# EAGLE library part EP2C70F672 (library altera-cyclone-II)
EP2C70F672 Auto generated by make-symbol-device-package-bsdl.ulp Rev. 19 Tip: Use split-device-symbol.ulp to generate a Device with multiple small symbols! Read HELP. Source: EP2C70F672.BSD
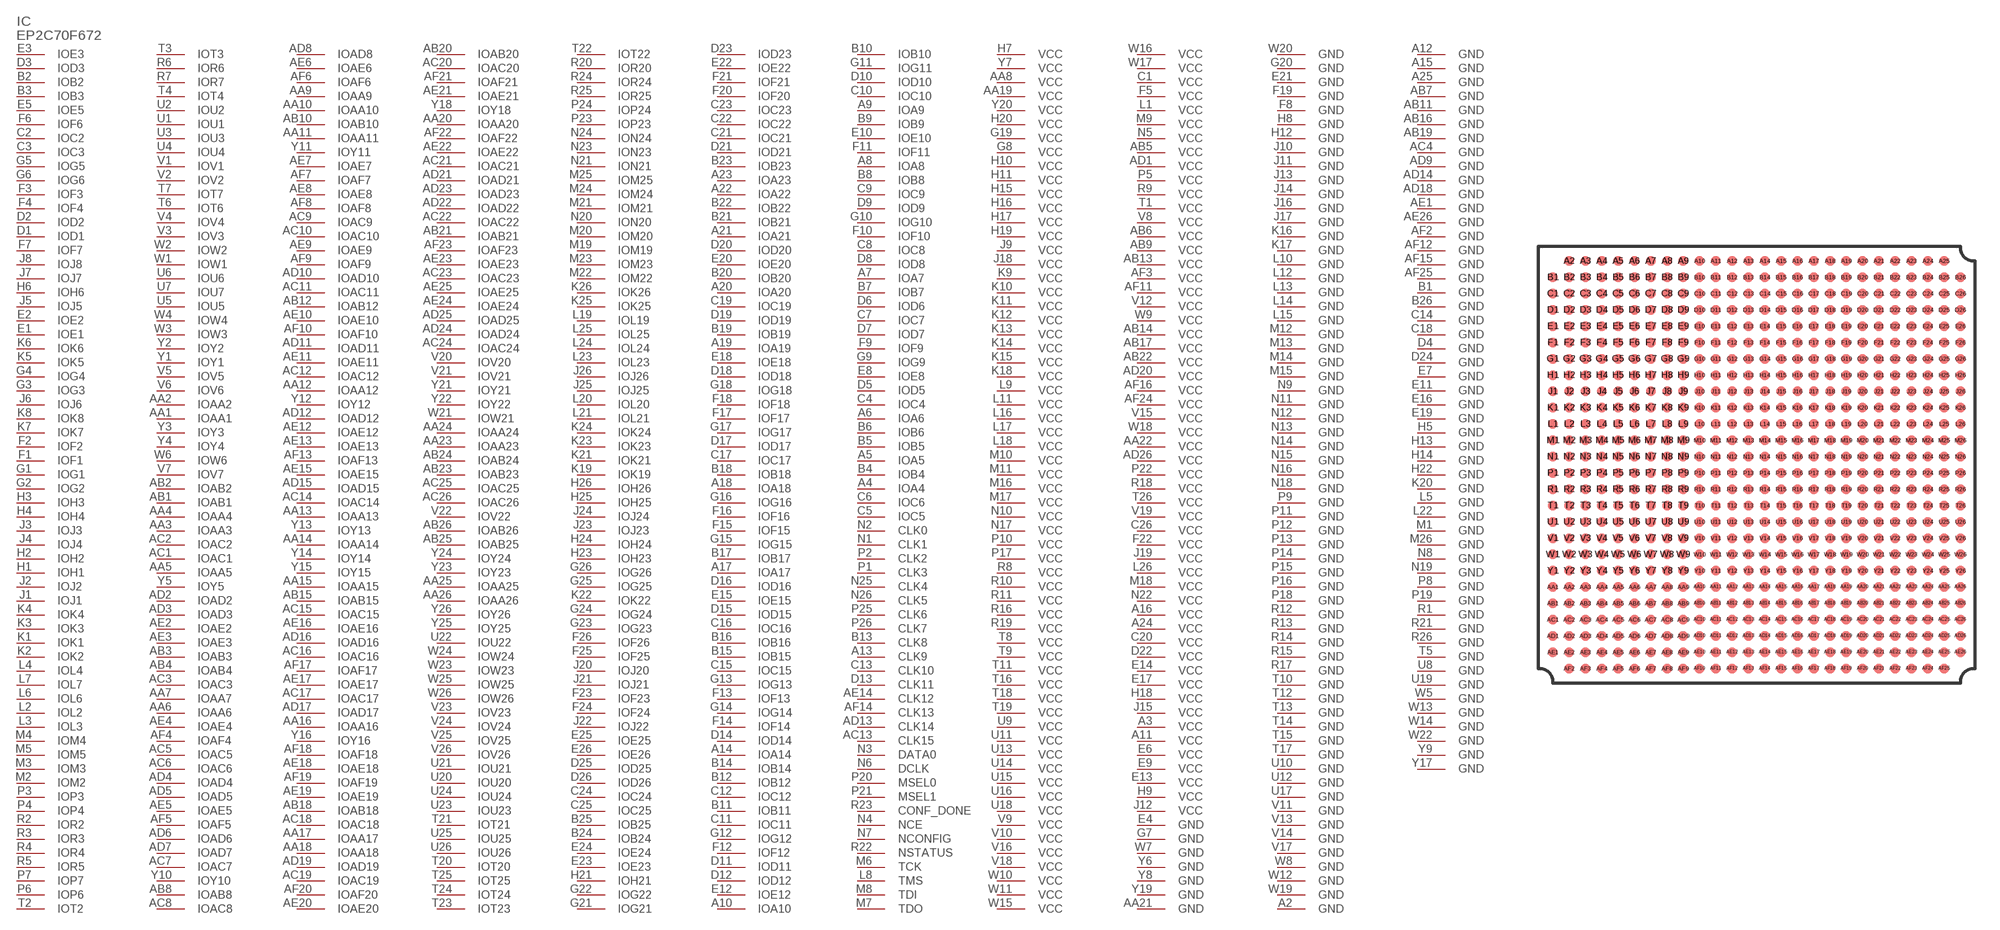
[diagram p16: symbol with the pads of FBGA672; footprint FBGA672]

Designator prefix IC

## EP2C70F672 (MPN: EP2C70F672C8N; OC_FARNELL: 1635091; OC_NEWARK: 51R0572)  [FBGA672]
A2  GND  pwr
A3  VCC  pwr
A4  IOA4
A5  IOA5
A6  IOA6
A7  IOA7
A8  IOA8
A9  IOA9
A10  IOA10
A11  VCC  pwr
A12  GND  pwr
A13  CLK9
A14  IOA14
A15  GND  pwr
A16  VCC  pwr
A17  IOA17
A18  IOA18
A19  IOA19
A20  IOA20
A21  IOA21
A22  IOA22
A23  IOA23
A24  VCC  pwr
A25  GND  pwr
AA1  IOAA1
AA2  IOAA2
AA3  IOAA3
AA4  IOAA4
AA5  IOAA5
AA6  IOAA6
AA7  IOAA7
AA8  VCC  pwr
AA9  IOAA9
AA10  IOAA10
AA11  IOAA11
AA12  IOAA12
AA13  IOAA13
AA14  IOAA14
AA15  IOAA15
AA16  IOAA16
AA17  IOAA17
AA18  IOAA18
AA19  VCC  pwr
AA20  IOAA20
AA21  GND  pwr
AA22  VCC  pwr
AA23  IOAA23
AA24  IOAA24
AA25  IOAA25
AA26  IOAA26
AB1  IOAB1
AB2  IOAB2
AB3  IOAB3
AB4  IOAB4
AB5  VCC  pwr
AB6  VCC  pwr
AB7  GND  pwr
AB8  IOAB8
AB9  VCC  pwr
AB10  IOAB10
AB11  GND  pwr
AB12  IOAB12
AB13  VCC  pwr
AB14  VCC  pwr
AB15  IOAB15
AB16  GND  pwr
AB17  VCC  pwr
AB18  IOAB18
AB19  GND  pwr
AB20  IOAB20
AB21  IOAB21
AB22  VCC  pwr
AB23  IOAB23
AB24  IOAB24
AB25  IOAB25
AB26  IOAB26
AC1  IOAC1
AC2  IOAC2
AC3  IOAC3
AC4  GND  pwr
AC5  IOAC5
AC6  IOAC6
AC7  IOAC7
AC8  IOAC8
AC9  IOAC9
AC10  IOAC10
AC11  IOAC11
AC12  IOAC12
AC13  CLK15
AC14  IOAC14
AC15  IOAC15
AC16  IOAC16
AC17  IOAC17
AC18  IOAC18
AC19  IOAC19
AC20  IOAC20
AC21  IOAC21
AC22  IOAC22
AC23  IOAC23
AC24  IOAC24
AC25  IOAC25
AC26  IOAC26
AD1  VCC  pwr
AD2  IOAD2
AD3  IOAD3
AD4  IOAD4
AD5  IOAD5
AD6  IOAD6
AD7  IOAD7
AD8  IOAD8
AD9  GND  pwr
AD10  IOAD10
AD11  IOAD11
AD12  IOAD12
AD13  CLK14
AD14  GND  pwr
AD15  IOAD15
AD16  IOAD16
AD17  IOAD17
AD18  GND  pwr
AD19  IOAD19
AD20  VCC  pwr
AD21  IOAD21
AD22  IOAD22
AD23  IOAD23
AD24  IOAD24
AD25  IOAD25
AD26  VCC  pwr
AE1  GND  pwr
AE2  IOAE2
AE3  IOAE3
AE4  IOAE4
AE5  IOAE5
AE6  IOAE6
AE7  IOAE7
AE8  IOAE8
AE9  IOAE9
AE10  IOAE10
AE11  IOAE11
AE12  IOAE12
AE13  IOAE13
AE14  CLK12
AE15  IOAE15
AE16  IOAE16
AE17  IOAE17
AE18  IOAE18
AE19  IOAE19
AE20  IOAE20
AE21  IOAE21
AE22  IOAE22
AE23  IOAE23
AE24  IOAE24
AE25  IOAE25
AE26  GND  pwr
AF2  GND  pwr
AF3  VCC  pwr
AF4  IOAF4
AF5  IOAF5
AF6  IOAF6
AF7  IOAF7
AF8  IOAF8
AF9  IOAF9
AF10  IOAF10
AF11  VCC  pwr
AF12  GND  pwr
AF13  IOAF13
AF14  CLK13
AF15  GND  pwr
AF16  VCC  pwr
AF17  IOAF17
AF18  IOAF18
AF19  IOAF19
AF20  IOAF20
AF21  IOAF21
AF22  IOAF22
AF23  IOAF23
AF24  VCC  pwr
AF25  GND  pwr
B1  GND  pwr
B2  IOB2
B3  IOB3
B4  IOB4
B5  IOB5
B6  IOB6
B7  IOB7
B8  IOB8
B9  IOB9
B10  IOB10
B11  IOB11
B12  IOB12
B13  CLK8
B14  IOB14
B15  IOB15
B16  IOB16
B17  IOB17
B18  IOB18
B19  IOB19
B20  IOB20
B21  IOB21
B22  IOB22
B23  IOB23
B24  IOB24
B25  IOB25
B26  GND  pwr
C1  VCC  pwr
C2  IOC2
C3  IOC3
C4  IOC4
C5  IOC5
C6  IOC6
C7  IOC7
C8  IOC8
C9  IOC9
C10  IOC10
C11  IOC11
C12  IOC12
C13  CLK10
C14  GND  pwr
C15  IOC15
C16  IOC16
C17  IOC17
C18  GND  pwr
C19  IOC19
C20  VCC  pwr
C21  IOC21
C22  IOC22
C23  IOC23
C24  IOC24
C25  IOC25
C26  VCC  pwr
D1  IOD1
D2  IOD2
D3  IOD3  out
D4  GND  pwr
D5  IOD5
D6  IOD6
D7  IOD7
D8  IOD8
D9  IOD9
D10  IOD10
D11  IOD11
D12  IOD12
D13  CLK11
D14  IOD14
D15  IOD15
D16  IOD16
D17  IOD17
D18  IOD18
D19  IOD19
D20  IOD20
D21  IOD21
D22  VCC  pwr
D23  IOD23
D24  GND  pwr
D25  IOD25
D26  IOD26
E1  IOE1
E2  IOE2
E3  IOE3  out
E4  GND  pwr
E5  IOE5
E6  VCC  pwr
E7  GND  pwr
E8  IOE8
E9  VCC  pwr
E10  IOE10
E11  GND  pwr
E12  IOE12
E13  VCC  pwr
E14  VCC  pwr
E15  IOE15
E16  GND  pwr
E17  VCC  pwr
E18  IOE18
E19  GND  pwr
E20  IOE20
E21  GND  pwr
E22  IOE22
E23  IOE23
E24  IOE24
E25  IOE25
E26  IOE26
F1  IOF1
F2  IOF2
F3  IOF3
F4  IOF4
F5  VCC  pwr
F6  IOF6
F7  IOF7
F8  GND  pwr
F9  IOF9
F10  IOF10
F11  IOF11
F12  IOF12
F13  IOF13
F14  IOF14
F15  IOF15
F16  IOF16
F17  IOF17
F18  IOF18
F19  GND  pwr
F20  IOF20
F21  IOF21
F22  VCC  pwr
F23  IOF23
F24  IOF24
F25  IOF25
F26  IOF26
G1  IOG1
G2  IOG2
G3  IOG3
G4  IOG4
G5  IOG5
G6  IOG6
G7  GND  pwr
G8  VCC  pwr
G9  IOG9
G10  IOG10
G11  IOG11
G12  IOG12
G13  IOG13
G14  IOG14
G15  IOG15
G16  IOG16
G17  IOG17
G18  IOG18
G19  VCC  pwr
G20  GND  pwr
G21  IOG21
G22  IOG22
G23  IOG23
G24  IOG24
G25  IOG25
G26  IOG26
H1  IOH1
H2  IOH2
H3  IOH3
H4  IOH4
H5  GND  pwr
H6  IOH6
H7  VCC  pwr
H8  GND  pwr
H9  VCC  pwr
H10  VCC  pwr
H11  VCC  pwr
H12  GND  pwr
H13  GND  pwr
H14  GND  pwr
H15  VCC  pwr
H16  VCC  pwr
H17  VCC  pwr
H18  VCC  pwr
H19  VCC  pwr
H20  VCC  pwr
H21  IOH21
H22  GND  pwr
H23  IOH23
H24  IOH24
H25  IOH25
H26  IOH26
J1  IOJ1
J2  IOJ2
J3  IOJ3
J4  IOJ4
J5  IOJ5
J6  IOJ6
J7  IOJ7
J8  IOJ8
J9  VCC  pwr
J10  GND  pwr
J11  GND  pwr
J12  VCC  pwr
J13  GND  pwr
J14  GND  pwr
J15  VCC  pwr
J16  GND  pwr
J17  GND  pwr
J18  VCC  pwr
J19  VCC  pwr
J20  IOJ20
J21  IOJ21
J22  IOJ22
J23  IOJ23
J24  IOJ24
J25  IOJ25
J26  IOJ26
K1  IOK1
K2  IOK2
K3  IOK3
K4  IOK4
K5  IOK5
K6  IOK6
K7  IOK7
K8  IOK8
K9  VCC  pwr
K10  VCC  pwr
K11  VCC  pwr
K12  VCC  pwr
K13  VCC  pwr
K14  VCC  pwr
K15  VCC  pwr
K16  GND  pwr
K17  GND  pwr
K18  VCC  pwr
K19  IOK19
K20  GND  pwr
K21  IOK21
K22  IOK22
K23  IOK23
K24  IOK24
K25  IOK25
K26  IOK26
L1  VCC  pwr
L2  IOL2
L3  IOL3
L4  IOL4
L5  GND  pwr
L6  IOL6
L7  IOL7
L8  TMS  in
L9  VCC  pwr
L10  GND  pwr
L11  VCC  pwr
L12  GND  pwr
L13  GND  pwr
L14  GND  pwr
L15  GND  pwr
L16  VCC  pwr
L17  VCC  pwr
L18  VCC  pwr
L19  IOL19
L20  IOL20
L21  IOL21
L22  GND  pwr
L23  IOL23
L24  IOL24
L25  IOL25
L26  VCC  pwr
M1  GND  pwr
M2  IOM2
M3  IOM3
M4  IOM4
M5  IOM5
M6  TCK  in
M7  TDO  out
M8  TDI  in
M9  VCC  pwr
M10  VCC  pwr
M11  VCC  pwr
M12  GND  pwr
M13  GND  pwr
M14  GND  pwr
M15  GND  pwr
M16  VCC  pwr
M17  VCC  pwr
M18  VCC  pwr
M19  IOM19
M20  IOM20
M21  IOM21
M22  IOM22
M23  IOM23
M24  IOM24
M25  IOM25
M26  GND  pwr
N1  CLK1
N2  CLK0
N3  DATA0
N4  NCE  in
N5  VCC  pwr
N6  DCLK
N7  NCONFIG  in
N8  GND  pwr
N9  GND  pwr
N10  VCC  pwr
N11  GND  pwr
N12  GND  pwr
N13  GND  pwr
N14  GND  pwr
N15  GND  pwr
N16  GND  pwr
N17  VCC  pwr
N18  GND  pwr
N19  GND  pwr
N20  ION20
N21  ION21
N22  VCC  pwr
N23  ION23
N24  ION24
N25  CLK4
N26  CLK5
P1  CLK3
P2  CLK2
P3  IOP3
P4  IOP4
P5  VCC  pwr
P6  IOP6
P7  IOP7
P8  GND  pwr
P9  GND  pwr
P10  VCC  pwr
P11  GND  pwr
P12  GND  pwr
P13  GND  pwr
P14  GND  pwr
P15  GND  pwr
P16  GND  pwr
P17  VCC  pwr
P18  GND  pwr
P19  GND  pwr
P20  MSEL0  in
P21  MSEL1  in
P22  VCC  pwr
P23  IOP23
P24  IOP24
P25  CLK6
P26  CLK7
R1  GND  pwr
R2  IOR2
R3  IOR3
R4  IOR4
R5  IOR5
R6  IOR6
R7  IOR7
R8  VCC  pwr
R9  VCC  pwr
R10  VCC  pwr
R11  VCC  pwr
R12  GND  pwr
R13  GND  pwr
R14  GND  pwr
R15  GND  pwr
R16  VCC  pwr
R17  GND  pwr
R18  VCC  pwr
R19  VCC  pwr
R20  IOR20
R21  GND  pwr
R22  NSTATUS  in
R23  CONF_DONE  in
R24  IOR24
R25  IOR25
R26  GND  pwr
T1  VCC  pwr
T2  IOT2
T3  IOT3
T4  IOT4
T5  GND  pwr
T6  IOT6
T7  IOT7
T8  VCC  pwr
T9  VCC  pwr
T10  GND  pwr
T11  VCC  pwr
T12  GND  pwr
T13  GND  pwr
T14  GND  pwr
T15  GND  pwr
T16  VCC  pwr
T17  GND  pwr
T18  VCC  pwr
T19  VCC  pwr
T20  IOT20
T21  IOT21
T22  IOT22
T23  IOT23
T24  IOT24
T25  IOT25
T26  VCC  pwr
U1  IOU1
U2  IOU2
U3  IOU3
U4  IOU4
U5  IOU5
U6  IOU6
U7  IOU7
U8  GND  pwr
U9  VCC  pwr
U10  GND  pwr
U11  VCC  pwr
U12  GND  pwr
U13  VCC  pwr
U14  VCC  pwr
U15  VCC  pwr
U16  VCC  pwr
U17  GND  pwr
U18  VCC  pwr
U19  GND  pwr
U20  IOU20
U21  IOU21
U22  IOU22
U23  IOU23
U24  IOU24
U25  IOU25
U26  IOU26
V1  IOV1
V2  IOV2
V3  IOV3
V4  IOV4
V5  IOV5
V6  IOV6
V7  IOV7
V8  VCC  pwr
V9  VCC  pwr
V10  VCC  pwr
V11  GND  pwr
V12  VCC  pwr
V13  GND  pwr
V14  GND  pwr
V15  VCC  pwr
V16  VCC  pwr
V17  GND  pwr
V18  VCC  pwr
V19  VCC  pwr
V20  IOV20
V21  IOV21
V22  IOV22
V23  IOV23
V24  IOV24
V25  IOV25
V26  IOV26
W1  IOW1
W2  IOW2
W3  IOW3
W4  IOW4
W5  GND  pwr
W6  IOW6
W7  GND  pwr
W8  GND  pwr
W9  VCC  pwr
W10  VCC  pwr
W11  VCC  pwr
W12  GND  pwr
W13  GND  pwr
W14  GND  pwr
W15  VCC  pwr
W16  VCC  pwr
W17  VCC  pwr
W18  VCC  pwr
W19  GND  pwr
W20  GND  pwr
W21  IOW21
W22  GND  pwr
W23  IOW23
W24  IOW24
W25  IOW25
W26  IOW26
Y1  IOY1
Y2  IOY2
Y3  IOY3
Y4  IOY4
Y5  IOY5
Y6  GND  pwr
Y7  VCC  pwr
Y8  GND  pwr
Y9  GND  pwr
Y10  IOY10
Y11  IOY11
Y12  IOY12
Y13  IOY13
Y14  IOY14
Y15  IOY15
Y16  IOY16
Y17  GND  pwr
Y18  IOY18
Y19  GND  pwr
Y20  VCC  pwr
Y21  IOY21
Y22  IOY22
Y23  IOY23
Y24  IOY24
Y25  IOY25
Y26  IOY26

## Footprint FBGA672 (pad centres in mm)
EP2C35F672 Auto generated by make-symbol-device-package-bsdl.ulp Rev. 19 Source: EP2C35F672.BSD www.altera.com .. cyc2_cii51015.pdf
smd 0.6 x 0.6: A2 -11.5,12.5; A3 -10.5,12.5; A4 -9.5,12.5; A5 -8.5,12.5; A6 -7.5,12.5; A7 -6.5,12.5; A8 -5.5,12.5; A9 -4.5,12.5; A10 -3.5,12.5; A11 -2.5,12.5; A12 -1.5,12.5; A13 -0.5,12.5; A14 0.5,12.5; A15 1.5,12.5; A16 2.5,12.5; A17 3.5,12.5; A18 4.5,12.5; A19 5.5,12.5; A20 6.5,12.5; A21 7.5,12.5; A22 8.5,12.5; A23 9.5,12.5; A24 10.5,12.5; A25 11.5,12.5; AA1 -12.5,-7.5; AA2 -11.5,-7.5; AA3 -10.5,-7.5; AA4 -9.5,-7.5; AA5 -8.5,-7.5; AA6 -7.5,-7.5; AA7 -6.5,-7.5; AA8 -5.5,-7.5; AA9 -4.5,-7.5; AA10 -3.5,-7.5; AA11 -2.5,-7.5; AA12 -1.5,-7.5; AA13 -0.5,-7.5; AA14 0.5,-7.5; AA15 1.5,-7.5; AA16 2.5,-7.5; AA17 3.5,-7.5; AA18 4.5,-7.5; AA19 5.5,-7.5; AA20 6.5,-7.5; AA21 7.5,-7.5; AA22 8.5,-7.5; AA23 9.5,-7.5; AA24 10.5,-7.5; AA25 11.5,-7.5; AA26 12.5,-7.5; AB1 -12.5,-8.5; AB2 -11.5,-8.5; AB3 -10.5,-8.5; AB4 -9.5,-8.5; AB5 -8.5,-8.5; AB6 -7.5,-8.5; AB7 -6.5,-8.5; AB8 -5.5,-8.5; AB9 -4.5,-8.5; AB10 -3.5,-8.5; AB11 -2.5,-8.5; AB12 -1.5,-8.5; AB13 -0.5,-8.5; AB14 0.5,-8.5; AB15 1.5,-8.5; AB16 2.5,-8.5; AB17 3.5,-8.5; AB18 4.5,-8.5; AB19 5.5,-8.5; AB20 6.5,-8.5; AB21 7.5,-8.5; AB22 8.5,-8.5; AB23 9.5,-8.5; AB24 10.5,-8.5; AB25 11.5,-8.5; AB26 12.5,-8.5; AC1 -12.5,-9.5; AC2 -11.5,-9.5; AC3 -10.5,-9.5; AC4 -9.5,-9.5; AC5 -8.5,-9.5; AC6 -7.5,-9.5; AC7 -6.5,-9.5; AC8 -5.5,-9.5; AC9 -4.5,-9.5; AC10 -3.5,-9.5; AC11 -2.5,-9.5; AC12 -1.5,-9.5; AC13 -0.5,-9.5; AC14 0.5,-9.5; AC15 1.5,-9.5; AC16 2.5,-9.5; AC17 3.5,-9.5; AC18 4.5,-9.5; AC19 5.5,-9.5; AC20 6.5,-9.5; AC21 7.5,-9.5; AC22 8.5,-9.5; AC23 9.5,-9.5; AC24 10.5,-9.5; AC25 11.5,-9.5; AC26 12.5,-9.5; AD1 -12.5,-10.5; AD2 -11.5,-10.5; AD3 -10.5,-10.5; AD4 -9.5,-10.5; AD5 -8.5,-10.5; AD6 -7.5,-10.5; AD7 -6.5,-10.5; AD8 -5.5,-10.5; AD9 -4.5,-10.5; AD10 -3.5,-10.5; AD11 -2.5,-10.5; AD12 -1.5,-10.5; AD13 -0.5,-10.5; AD14 0.5,-10.5; AD15 1.5,-10.5; AD16 2.5,-10.5; AD17 3.5,-10.5; AD18 4.5,-10.5; AD19 5.5,-10.5; AD20 6.5,-10.5; AD21 7.5,-10.5; AD22 8.5,-10.5; AD23 9.5,-10.5; AD24 10.5,-10.5; AD25 11.5,-10.5; AD26 12.5,-10.5; AE1 -12.5,-11.5; AE2 -11.5,-11.5; AE3 -10.5,-11.5; AE4 -9.5,-11.5; AE5 -8.5,-11.5; AE6 -7.5,-11.5; AE7 -6.5,-11.5; AE8 -5.5,-11.5; AE9 -4.5,-11.5; AE10 -3.5,-11.5; AE11 -2.5,-11.5; AE12 -1.5,-11.5; AE13 -0.5,-11.5; AE14 0.5,-11.5; AE15 1.5,-11.5; AE16 2.5,-11.5; AE17 3.5,-11.5; AE18 4.5,-11.5; AE19 5.5,-11.5; AE20 6.5,-11.5; AE21 7.5,-11.5; AE22 8.5,-11.5; AE23 9.5,-11.5; AE24 10.5,-11.5; AE25 11.5,-11.5; AE26 12.5,-11.5; AF2 -11.5,-12.5; AF3 -10.5,-12.5; AF4 -9.5,-12.5; AF5 -8.5,-12.5; AF6 -7.5,-12.5; AF7 -6.5,-12.5; AF8 -5.5,-12.5; AF9 -4.5,-12.5; AF10 -3.5,-12.5; AF11 -2.5,-12.5; AF12 -1.5,-12.5; AF13 -0.5,-12.5; AF14 0.5,-12.5; AF15 1.5,-12.5; AF16 2.5,-12.5; AF17 3.5,-12.5; AF18 4.5,-12.5; AF19 5.5,-12.5; AF20 6.5,-12.5; AF21 7.5,-12.5; AF22 8.5,-12.5; AF23 9.5,-12.5; AF24 10.5,-12.5; AF25 11.5,-12.5; B1 -12.5,11.5; B2 -11.5,11.5; B3 -10.5,11.5; B4 -9.5,11.5; B5 -8.5,11.5; B6 -7.5,11.5; B7 -6.5,11.5; B8 -5.5,11.5; B9 -4.5,11.5; B10 -3.5,11.5; B11 -2.5,11.5; B12 -1.5,11.5; B13 -0.5,11.5; B14 0.5,11.5; B15 1.5,11.5; B16 2.5,11.5; B17 3.5,11.5; B18 4.5,11.5; B19 5.5,11.5; B20 6.5,11.5; B21 7.5,11.5; B22 8.5,11.5; B23 9.5,11.5; B24 10.5,11.5; B25 11.5,11.5; B26 12.5,11.5; C1 -12.5,10.5; C2 -11.5,10.5; C3 -10.5,10.5; C4 -9.5,10.5; C5 -8.5,10.5; C6 -7.5,10.5; C7 -6.5,10.5; C8 -5.5,10.5; C9 -4.5,10.5; C10 -3.5,10.5; C11 -2.5,10.5; C12 -1.5,10.5; C13 -0.5,10.5; C14 0.5,10.5; C15 1.5,10.5; C16 2.5,10.5; C17 3.5,10.5; C18 4.5,10.5; C19 5.5,10.5; C20 6.5,10.5; C21 7.5,10.5; C22 8.5,10.5; C23 9.5,10.5; C24 10.5,10.5; C25 11.5,10.5; C26 12.5,10.5; D1 -12.5,9.5; D2 -11.5,9.5; D3 -10.5,9.5; D4 -9.5,9.5; D5 -8.5,9.5; D6 -7.5,9.5; D7 -6.5,9.5; D8 -5.5,9.5; D9 -4.5,9.5; D10 -3.5,9.5; D11 -2.5,9.5; D12 -1.5,9.5; D13 -0.5,9.5; D14 0.5,9.5; D15 1.5,9.5; D16 2.5,9.5; D17 3.5,9.5; D18 4.5,9.5; D19 5.5,9.5; D20 6.5,9.5; D21 7.5,9.5; D22 8.5,9.5; D23 9.5,9.5; D24 10.5,9.5; D25 11.5,9.5; D26 12.5,9.5; E1 -12.5,8.5; E2 -11.5,8.5; E3 -10.5,8.5; E4 -9.5,8.5; E5 -8.5,8.5; E6 -7.5,8.5; E7 -6.5,8.5; E8 -5.5,8.5; E9 -4.5,8.5; E10 -3.5,8.5; E11 -2.5,8.5; E12 -1.5,8.5; E13 -0.5,8.5; E14 0.5,8.5; E15 1.5,8.5; E16 2.5,8.5; E17 3.5,8.5; E18 4.5,8.5; E19 5.5,8.5; E20 6.5,8.5; E21 7.5,8.5; E22 8.5,8.5; E23 9.5,8.5; E24 10.5,8.5; E25 11.5,8.5; E26 12.5,8.5; F1 -12.5,7.5; F2 -11.5,7.5; F3 -10.5,7.5; F4 -9.5,7.5; F5 -8.5,7.5; F6 -7.5,7.5; F7 -6.5,7.5; F8 -5.5,7.5; F9 -4.5,7.5; F10 -3.5,7.5; F11 -2.5,7.5; F12 -1.5,7.5; F13 -0.5,7.5; F14 0.5,7.5; F15 1.5,7.5; F16 2.5,7.5; F17 3.5,7.5; F18 4.5,7.5; F19 5.5,7.5; F20 6.5,7.5; F21 7.5,7.5; F22 8.5,7.5; F23 9.5,7.5; F24 10.5,7.5; F25 11.5,7.5; F26 12.5,7.5; G1 -12.5,6.5; G2 -11.5,6.5; G3 -10.5,6.5; G4 -9.5,6.5; G5 -8.5,6.5; G6 -7.5,6.5; G7 -6.5,6.5; G8 -5.5,6.5; G9 -4.5,6.5; G10 -3.5,6.5; G11 -2.5,6.5; G12 -1.5,6.5; G13 -0.5,6.5; G14 0.5,6.5; G15 1.5,6.5; G16 2.5,6.5; G17 3.5,6.5; G18 4.5,6.5; G19 5.5,6.5; G20 6.5,6.5; G21 7.5,6.5; G22 8.5,6.5; G23 9.5,6.5; G24 10.5,6.5; G25 11.5,6.5; G26 12.5,6.5; H1 -12.5,5.5; H2 -11.5,5.5; H3 -10.5,5.5; H4 -9.5,5.5; H5 -8.5,5.5; H6 -7.5,5.5; H7 -6.5,5.5; H8 -5.5,5.5; H9 -4.5,5.5; H10 -3.5,5.5; H11 -2.5,5.5; H12 -1.5,5.5; H13 -0.5,5.5; H14 0.5,5.5; H15 1.5,5.5; H16 2.5,5.5; H17 3.5,5.5; H18 4.5,5.5; H19 5.5,5.5; H20 6.5,5.5; H21 7.5,5.5; H22 8.5,5.5; H23 9.5,5.5; H24 10.5,5.5; H25 11.5,5.5; H26 12.5,5.5; J1 -12.5,4.5; J2 -11.5,4.5; J3 -10.5,4.5; J4 -9.5,4.5; J5 -8.5,4.5; J6 -7.5,4.5; J7 -6.5,4.5; J8 -5.5,4.5; J9 -4.5,4.5; J10 -3.5,4.5; J11 -2.5,4.5; J12 -1.5,4.5; J13 -0.5,4.5; J14 0.5,4.5; J15 1.5,4.5; J16 2.5,4.5; J17 3.5,4.5; J18 4.5,4.5; J19 5.5,4.5; J20 6.5,4.5; J21 7.5,4.5; J22 8.5,4.5; J23 9.5,4.5; J24 10.5,4.5; J25 11.5,4.5; J26 12.5,4.5; K1 -12.5,3.5; K2 -11.5,3.5; K3 -10.5,3.5; K4 -9.5,3.5; K5 -8.5,3.5; K6 -7.5,3.5; K7 -6.5,3.5; K8 -5.5,3.5; K9 -4.5,3.5; K10 -3.5,3.5; K11 -2.5,3.5; K12 -1.5,3.5; K13 -0.5,3.5; K14 0.5,3.5; K15 1.5,3.5; K16 2.5,3.5; K17 3.5,3.5; K18 4.5,3.5; K19 5.5,3.5; K20 6.5,3.5; K21 7.5,3.5; K22 8.5,3.5; K23 9.5,3.5; K24 10.5,3.5; K25 11.5,3.5; K26 12.5,3.5; L1 -12.5,2.5; L2 -11.5,2.5; L3 -10.5,2.5; L4 -9.5,2.5; L5 -8.5,2.5; L6 -7.5,2.5; L7 -6.5,2.5; L8 -5.5,2.5; L9 -4.5,2.5; L10 -3.5,2.5; L11 -2.5,2.5; L12 -1.5,2.5; L13 -0.5,2.5; L14 0.5,2.5; L15 1.5,2.5; L16 2.5,2.5; L17 3.5,2.5; L18 4.5,2.5; L19 5.5,2.5; L20 6.5,2.5; L21 7.5,2.5; L22 8.5,2.5; L23 9.5,2.5; L24 10.5,2.5; L25 11.5,2.5; L26 12.5,2.5; M1 -12.5,1.5; M2 -11.5,1.5; M3 -10.5,1.5; M4 -9.5,1.5; M5 -8.5,1.5; M6 -7.5,1.5; M7 -6.5,1.5; M8 -5.5,1.5; M9 -4.5,1.5; M10 -3.5,1.5; M11 -2.5,1.5; M12 -1.5,1.5; M13 -0.5,1.5; M14 0.5,1.5; M15 1.5,1.5; M16 2.5,1.5; M17 3.5,1.5; M18 4.5,1.5; M19 5.5,1.5; M20 6.5,1.5; M21 7.5,1.5; M22 8.5,1.5; M23 9.5,1.5; M24 10.5,1.5; M25 11.5,1.5; M26 12.5,1.5; N1 -12.5,0.5; N2 -11.5,0.5; N3 -10.5,0.5; N4 -9.5,0.5; N5 -8.5,0.5; N6 -7.5,0.5; N7 -6.5,0.5; N8 -5.5,0.5; N9 -4.5,0.5; N10 -3.5,0.5; N11 -2.5,0.5; N12 -1.5,0.5; N13 -0.5,0.5; N14 0.5,0.5; N15 1.5,0.5; N16 2.5,0.5; N17 3.5,0.5; N18 4.5,0.5; N19 5.5,0.5; N20 6.5,0.5; N21 7.5,0.5; N22 8.5,0.5; N23 9.5,0.5; N24 10.5,0.5; N25 11.5,0.5; N26 12.5,0.5; P1 -12.5,-0.5; P2 -11.5,-0.5; P3 -10.5,-0.5; P4 -9.5,-0.5; P5 -8.5,-0.5; P6 -7.5,-0.5; P7 -6.5,-0.5; P8 -5.5,-0.5; P9 -4.5,-0.5; P10 -3.5,-0.5; P11 -2.5,-0.5; P12 -1.5,-0.5; P13 -0.5,-0.5; P14 0.5,-0.5; P15 1.5,-0.5; P16 2.5,-0.5; P17 3.5,-0.5; P18 4.5,-0.5; P19 5.5,-0.5; P20 6.5,-0.5; P21 7.5,-0.5; P22 8.5,-0.5; P23 9.5,-0.5; P24 10.5,-0.5; P25 11.5,-0.5; P26 12.5,-0.5; R1 -12.5,-1.5; R2 -11.5,-1.5; R3 -10.5,-1.5; R4 -9.5,-1.5; R5 -8.5,-1.5; R6 -7.5,-1.5; R7 -6.5,-1.5; R8 -5.5,-1.5; R9 -4.5,-1.5; R10 -3.5,-1.5; R11 -2.5,-1.5; R12 -1.5,-1.5; R13 -0.5,-1.5; R14 0.5,-1.5; R15 1.5,-1.5; R16 2.5,-1.5; R17 3.5,-1.5; R18 4.5,-1.5; R19 5.5,-1.5; R20 6.5,-1.5; R21 7.5,-1.5; R22 8.5,-1.5; R23 9.5,-1.5; R24 10.5,-1.5; R25 11.5,-1.5; R26 12.5,-1.5; T1 -12.5,-2.5; T2 -11.5,-2.5; T3 -10.5,-2.5; T4 -9.5,-2.5; T5 -8.5,-2.5; T6 -7.5,-2.5; T7 -6.5,-2.5; T8 -5.5,-2.5; T9 -4.5,-2.5; T10 -3.5,-2.5; T11 -2.5,-2.5; T12 -1.5,-2.5; T13 -0.5,-2.5; T14 0.5,-2.5; T15 1.5,-2.5; T16 2.5,-2.5; T17 3.5,-2.5; T18 4.5,-2.5; T19 5.5,-2.5; T20 6.5,-2.5; T21 7.5,-2.5; T22 8.5,-2.5; T23 9.5,-2.5; T24 10.5,-2.5; T25 11.5,-2.5; T26 12.5,-2.5; U1 -12.5,-3.5; U2 -11.5,-3.5; U3 -10.5,-3.5; U4 -9.5,-3.5; U5 -8.5,-3.5; U6 -7.5,-3.5; U7 -6.5,-3.5; U8 -5.5,-3.5; U9 -4.5,-3.5; U10 -3.5,-3.5; U11 -2.5,-3.5; U12 -1.5,-3.5; U13 -0.5,-3.5; U14 0.5,-3.5; U15 1.5,-3.5; U16 2.5,-3.5; U17 3.5,-3.5; U18 4.5,-3.5; U19 5.5,-3.5; U20 6.5,-3.5; U21 7.5,-3.5; U22 8.5,-3.5; U23 9.5,-3.5; U24 10.5,-3.5; U25 11.5,-3.5; U26 12.5,-3.5; V1 -12.5,-4.5; V2 -11.5,-4.5; V3 -10.5,-4.5; V4 -9.5,-4.5; V5 -8.5,-4.5; V6 -7.5,-4.5; V7 -6.5,-4.5; V8 -5.5,-4.5; V9 -4.5,-4.5; V10 -3.5,-4.5; V11 -2.5,-4.5; V12 -1.5,-4.5; V13 -0.5,-4.5; V14 0.5,-4.5; V15 1.5,-4.5; V16 2.5,-4.5; V17 3.5,-4.5; V18 4.5,-4.5; V19 5.5,-4.5; V20 6.5,-4.5; V21 7.5,-4.5; V22 8.5,-4.5; V23 9.5,-4.5; V24 10.5,-4.5; V25 11.5,-4.5; V26 12.5,-4.5; W1 -12.5,-5.5; W2 -11.5,-5.5; W3 -10.5,-5.5; W4 -9.5,-5.5; W5 -8.5,-5.5; W6 -7.5,-5.5; W7 -6.5,-5.5; W8 -5.5,-5.5; W9 -4.5,-5.5; W10 -3.5,-5.5; W11 -2.5,-5.5; W12 -1.5,-5.5; W13 -0.5,-5.5; W14 0.5,-5.5; W15 1.5,-5.5; W16 2.5,-5.5; W17 3.5,-5.5; W18 4.5,-5.5; W19 5.5,-5.5; W20 6.5,-5.5; W21 7.5,-5.5; W22 8.5,-5.5; W23 9.5,-5.5; W24 10.5,-5.5; W25 11.5,-5.5; W26 12.5,-5.5; Y1 -12.5,-6.5; Y2 -11.5,-6.5; Y3 -10.5,-6.5; Y4 -9.5,-6.5; Y5 -8.5,-6.5; Y6 -7.5,-6.5; Y7 -6.5,-6.5; Y8 -5.5,-6.5; Y9 -4.5,-6.5; Y10 -3.5,-6.5; Y11 -2.5,-6.5; Y12 -1.5,-6.5; Y13 -0.5,-6.5; Y14 0.5,-6.5; Y15 1.5,-6.5; Y16 2.5,-6.5; Y17 3.5,-6.5; Y18 4.5,-6.5; Y19 5.5,-6.5; Y20 6.5,-6.5; Y21 7.5,-6.5; Y22 8.5,-6.5; Y23 9.5,-6.5; Y24 10.5,-6.5; Y25 11.5,-6.5; Y26 12.5,-6.5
